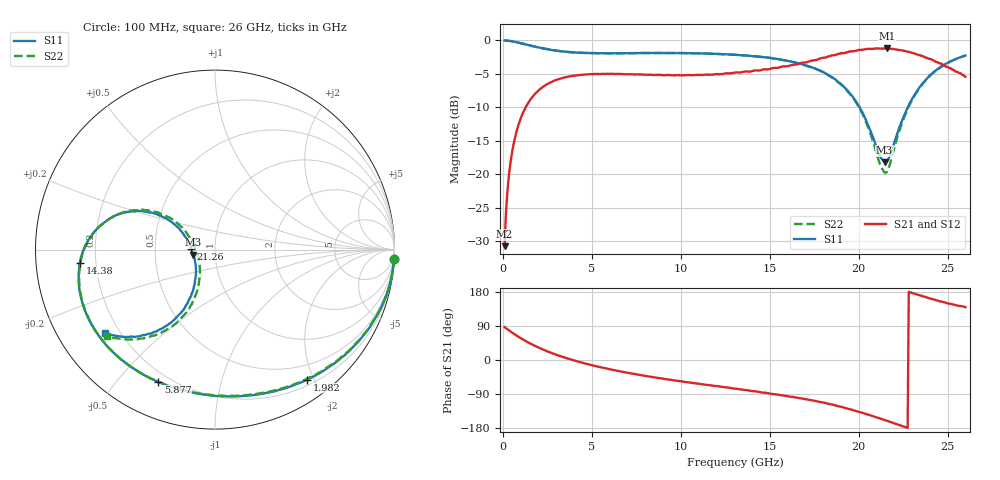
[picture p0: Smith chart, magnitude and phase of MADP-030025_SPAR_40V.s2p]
!Mean
# HZ S DB R 50
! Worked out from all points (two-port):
!   400 points, 100 MHz to 26 GHz, reference 50 ohm
!   highest |S21| = -1.18 dB at 21.59 GHz (marker M1); lowest = -30.7 dB at 100 MHz (marker M2)
!   |S21| within 3 dB of the highest: 15.12 GHz to 25.19 GHz (10.07 GHz wide, 50 % of centre)
!   lowest |S11| = -18.2 dB at 21.46 GHz (marker M3), VSWR 1.28, Z = 39.2 - j2.26 ohm
!   |S11| at or under -10 dB: 20.06 GHz to 22.76 GHz (2.703 GHz wide, 12.6 % of centre)
!   |S22| runs from -19.8 to 0.0 dB; largest |S21 - S12| = 0.0082
!   S11 on the Smith chart (normalised r, x): 100 MHz: 2, -37; 1.982 GHz: 0.28, -1.90; 5.877 GHz: 0.16, -0.65; 14.38 GHz: 0.14, -0.05; 21.26 GHz: 0.77, +0.01; 26 GHz: 0.14, -0.33
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1e8  -0.02 -3.1  -30.73 86.7  -30.76 86.6  -0.00 -3.1
1.6491e8  -0.03 -4.9  -26.39 84.3  -26.42 84.4  -0.00 -5.1
2.9474e8  -0.04 -9.3  -21.44 79.8  -21.43 79.6  -0.04 -9.2
6.193e8  -0.17 -19.3  -15.30 69.2  -15.30 69.2  -0.17 -18.9
1.1386e9  -0.50 -34.1  -10.78 53.8  -10.78 53.8  -0.50 -33.4
1.9825e9  -1.03 -54.7  -7.52 33.4  -7.52 33.4  -1.04 -53.4
3.086e9  -1.55 -76.2  -5.83 12.5  -5.81 12.5  -1.56 -74.5
4.4491e9  -1.84 -96.6  -5.13 -7.1  -5.12 -7.1  -1.86 -94.7
5.8772e9  -1.92 -113.2  -4.98 -23.1  -4.99 -23.2  -1.93 -111.4
8.7982e9  -1.87 -138.6  -5.13 -47.7  -5.14 -47.8  -1.88 -137.2
1.3082e10  -2.15 -166.5  -4.80 -75.7  -4.81 -75.7  -2.15 -165.8
1.4381e10  -2.42 -174.3  -4.48 -84.2  -4.49 -84.2  -2.43 -173.8
1.7367e10  -4.01 165.7  -3.01 -106.3  -3.03 -106.2  -4.03 165.5
1.9704e10  -8.57 148.6  -1.64 -132.5  -1.64 -132.7  -8.64 146.7
2.1261e10  -17.58 177.6  -1.21 -155.1  -1.22 -155.2  -18.82 175.0
2.1456e10  -18.18 -166.7  -1.21 -158.2  -1.21 -158.2  -19.72 -167.1
2.1586e10  -18.10 -155.2  -1.18 -160.3  -1.18 -160.2  -19.66 -152.5
2.1716e10  -17.47 -144.4  -1.22 -162.5  -1.23 -162.4  -18.84 -139.8
2.2625e10  -10.79 -117.2  -1.58 -177.0  -1.58 -176.9  -11.01 -113.0
2.3404e10  -7.08 -119.9  -2.18 171.0  -2.16 171.0  -7.18 -116.8
2.4572e10  -4.05 -130.4  -3.41 154.4  -3.39 154.9  -4.09 -128.3
2.6e10  -2.25 -142.8  -5.42 139.3  -5.31 139.4  -2.26 -141.3
